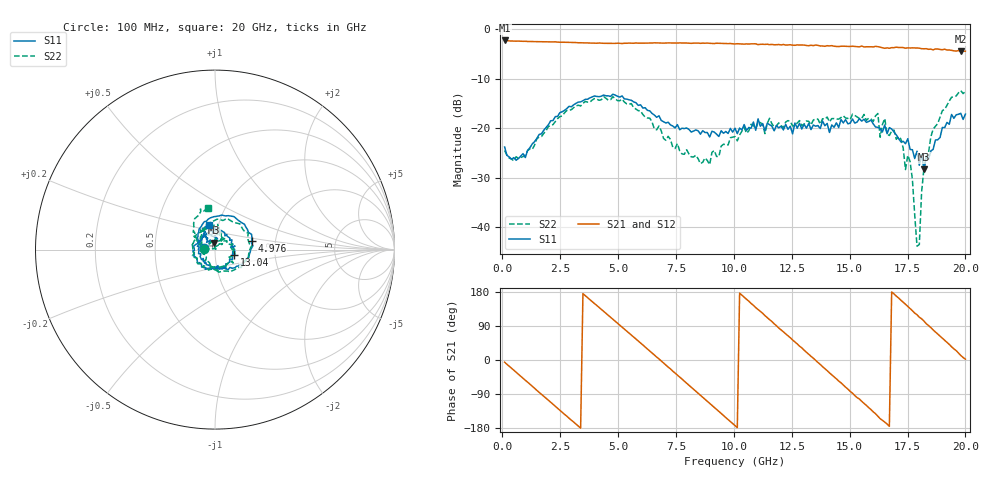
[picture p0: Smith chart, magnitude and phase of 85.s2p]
!Agilent Technologies,N5230C,MY49001569,A.09.33.09
!Agilent N5230C: A.09.33.09
!Date: Tuesday, July 28, 2015 17:42:14
!Correction: S11(Full 2 Port(1,2))
!S21(Full 2 Port(1,2))
!S12(Full 2 Port(1,2))
!S22(Full 2 Port(1,2))
!S2P File: Measurements: S11, S21, S12, S22:
# Hz S  dB  R 50
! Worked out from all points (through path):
!   201 points, 100 MHz to 20 GHz, reference 50 ohm
!   highest |S21| = -2.28 dB at 100 MHz (marker M1); lowest = -4.5 dB at 19.8 GHz (marker M2)
!   group delay of S21, straight-line fit = 149 ps
!   lowest |S11| = -28.3 dB at 18.21 GHz (marker M3), VSWR 1.08, Z = 49.3 + j3.77 ohm
!   |S11| at or under -10 dB: start of sweep to end of sweep
!   |S22| runs from -43.8 to -12.4 dB; largest |S21 - S12| = 0.02
!   S11 on the Smith chart (normalised r, x): 100 MHz: 0.88, +0.02; 4.976 GHz: 1.51, +0.15; 13.04 GHz: 1.23, -0.08; 20 GHz: 0.91, +0.25
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1e8  -23.77 170.2  -2.28 -5.7  -2.26 -6.0  -24.48 174.3
9.955e8  -25.90 173.3  -2.45 -53.5  -2.49 -53.6  -25.38 163.8
1.7915e9  -20.38 157.7  -2.55 -95.9  -2.56 -96.0  -21.02 147.4
2.687e9  -16.38 119.6  -2.64 -143.3  -2.70 -143.3  -16.88 110.0
3.483e9  -14.44 82.7  -2.76 175.1  -2.78 174.9  -14.97 71.1
4.9755e9  -13.54 13.4  -2.83 97.2  -2.85 97.2  -14.42 -3.1
5.7715e9  -14.83 -19.4  -2.79 55.4  -2.81 55.4  -16.11 -45.7
6.7665e9  -17.48 -56.3  -2.77 2.8  -2.79 2.6  -19.54 -105.5
8.458e9  -20.50 -120.8  -2.80 -87.5  -2.86 -88.0  -26.16 141.7
1.005e10  -19.98 154.2  -2.99 -173.1  -2.94 -173.2  -21.68 35.3
1.1642e10  -19.55 58.2  -3.08 101.7  -3.02 102.0  -19.08 -36.0
1.3035e10  -19.19 -16.5  -3.21 25.9  -3.28 25.4  -19.14 -125.9
1.3433e10  -19.34 -39.9  -3.33 4.8  -3.25 3.9  -18.34 -138.8
1.51245e10  -18.13 -140.8  -3.44 -87.6  -3.47 -87.4  -17.15 147.8
1.67165e10  -19.86 125.1  -3.86 -175.0  -3.74 -174.8  -21.44 71.8
1.7612e10  -24.27 76.2  -3.80 135.4  -3.89 135.3  -26.69 36.7
1.79105e10  -24.61 89.9  -3.80 119.4  -3.83 118.9  -43.77 25.5
1.801e10  -27.45 81.8  -3.83 112.9  -3.96 113.2  -43.43 74.8
1.8209e10  -28.26 98.3  -3.96 102.9  -3.96 101.4  -28.15 174.6
1.8607e10  -24.25 139.5  -4.18 79.4  -3.91 79.4  -20.14 158.8
1.9801e10  -16.97 109.7  -4.47 12.1  -4.39 12.3  -12.40 109.9
2e10  -17.14 102.9  -4.46 2.2  -4.63 1.2  -12.59 99.3
